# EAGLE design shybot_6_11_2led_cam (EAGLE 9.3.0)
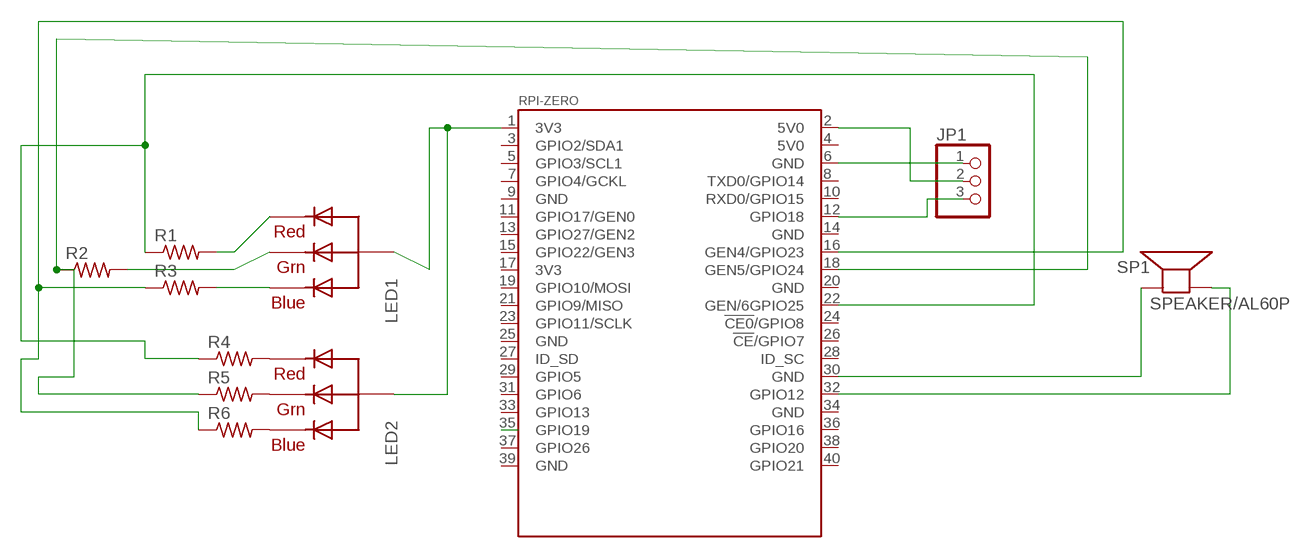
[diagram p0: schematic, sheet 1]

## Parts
JP1  PINHD-1X3  [1X03]
LED1  RGBLED_CA-5MM  [LED5MMRGB]
LED2  RGBLED_CA-5MM  [LED5MMRGB]
R1  R-US_0204/7  [0204/7]
R2  R-US_0204/7  [0204/7]
R3  R-US_0204/7  [0204/7]
R4  R-US_0204/7  [0204/7]
R5  R-US_0204/7  [0204/7]
R6  R-US_0204/7  [0204/7]
SP1  SPEAKER/AL60P  [AL60P]
U$1  RPI-ZERO  [RASPBERRYPI_BASTELSTUBE_V13_RASPI_BOARD_B+_FULL]

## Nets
3V3@1: LED1.2(VCC) LED2.2(VCC) U$1.1(3V3)
5V0@1: JP1.2 U$1.2(5V0)
GND@6: SP1.1(+) U$1.30(GND)
GND@8: JP1.1 U$1.6(GND)
N$1: JP1.3 U$1.12(GPIO18)
N$2: LED1.1(RED) R1.2
N$3: LED1.3(GREEN) R2.2
N$4: LED1.4(BLUE) R3.2
N$5: R2.1 R5.1 U$1.18(GEN5/GPIO24)
N$6: R1.1 R4.1 U$1.22(GEN/6GPIO25)
N$7: R3.1 R6.1 U$1.16(GEN4/GPIO23)
N$8: SP1.2(-) U$1.32(GPIO12)
N$9: LED2.1(RED) R4.2
N$10: U$1.35(GPIO19)
N$11: LED2.3(GREEN) R5.2
N$12: LED2.4(BLUE) R6.2
Unconnected: U$1.3(GPIO2/SDA1) U$1.4(5V0) U$1.5(GPIO3/SCL1) U$1.7(GPIO4/GCKL) U$1.8(TXD0/GPIO14) U$1.9(GND) U$1.10(RXD0/GPIO15) U$1.11(GPIO17/GEN0) U$1.13(GPIO27/GEN2) U$1.14(GND) U$1.15(GPIO22/GEN3) U$1.17(3V3) U$1.19(GPIO10/MOSI) U$1.20(GND) U$1.21(GPIO9/MISO) U$1.23(GPIO11/SCLK) U$1.24(!CE0!/GPIO8) U$1.25(GND) U$1.26(!CE!/GPIO7) U$1.27(ID_SD) U$1.28(ID_SC) U$1.29(GPIO5) U$1.31(GPIO6) U$1.33(GPIO13) U$1.34(GND) U$1.36(GPIO16) U$1.37(GPIO26) U$1.38(GPIO20) U$1.39(GND) U$1.40(GPIO21)

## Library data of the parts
JP1 = pinhead:PINHD-1X3: PIN HEADER
LED1 LED2 = adafruit:RGBLED_CA: RGB LED, common-anode 5MM Staggered pins 5mm Piranha package http://www.ladyada.net/library/pcb/eaglelibrary.html
R1-R6 = adafruit:R-US_: RESISTOR, American symbol
SP1 = adafruit:SPEAKER: SPEAKER
U$1 = RPI-Zero:RPI-ZERO

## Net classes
0 default: width 0.381 mm, drill 0.533 mm, clearance 0.406 mm

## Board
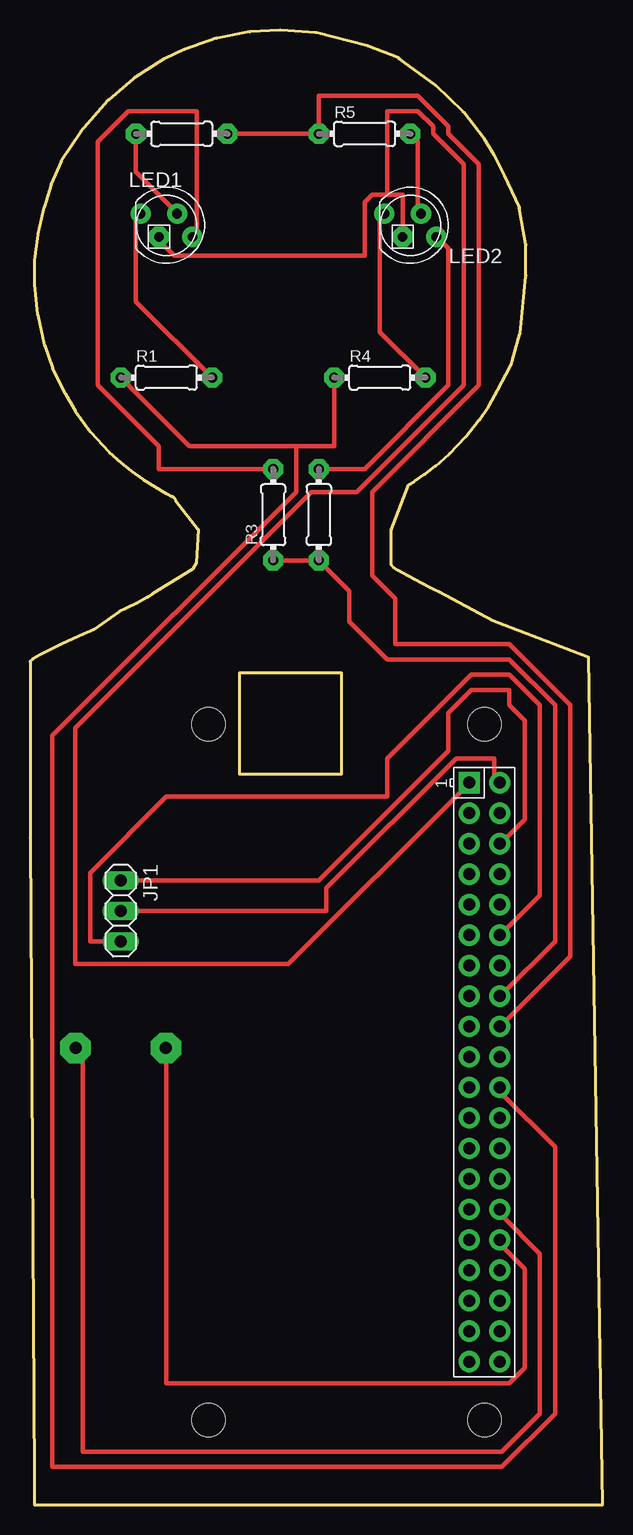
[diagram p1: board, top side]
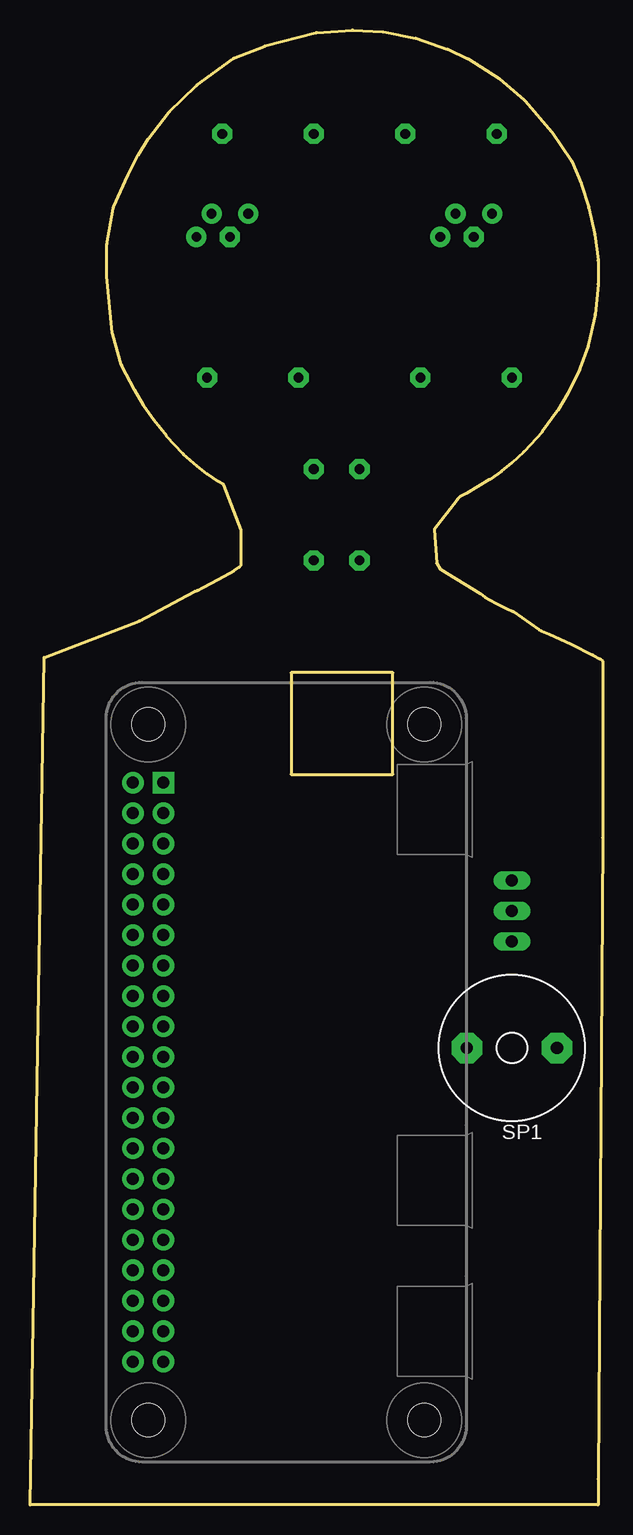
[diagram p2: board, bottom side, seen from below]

Size 47.72 x 122.96 mm. Coordinates in mm from the lower left corner, seen from the top.
Outline: 126 segments
Copper layers (1*16): Top 0.035mm / dielectric 1.5mm / Bottom 0.035mm
Design rules "default": minimum track width 6mil, minimum drill 0.35mm, track to track 6mil, track to pad 6mil, pad to pad 6mil, via to via 6mil, smd to smd 6mil, copper to edge 40mil, drill to drill 6mil, minimum pad ring 10mil, minimum via ring 8mil, stop-mask expansion 4mil, vias tented up to drill 0mil, thermal gap 10mil

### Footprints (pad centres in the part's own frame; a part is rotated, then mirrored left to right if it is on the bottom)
1X03 = drill 1.016 long: 1 -2.54,0; 2 0,0; 3 2.54,0
LED5MMRGB = drill 0.8 pad 1.676: 1 -2.159,0.968; 3 0.889,0.968; 4 2.159,-0.968 | drill 0.8 pad 1.676 octagon: 2 -0.635,-0.968
0204/7 = drill 0.813 pad 1.676 octagon: 1 -3.81,0; 2 3.81,0
AL60P = drill 1.016 pad 2.54 octagon: 1 -3.759,0; 2 3.759,0
RASPBERRYPI_BASTELSTUBE_V13_RASPI_BOARD_B+_FULL = drill 1 pad 1.778 square: 1 8.37,25.23 | drill 1 pad 1.778: 2 8.37,27.77; 3 10.91,25.23; 4 10.91,27.77; 5 13.45,25.23; 6 13.45,27.77; 7 15.99,25.23; 8 15.99,27.77; 9 18.53,25.23; 10 18.53,27.77; 11 21.07,25.23; 12 21.07,27.77; 13 23.61,25.23; 14 23.61,27.77; 15 26.15,25.23; 16 26.15,27.77; 17 28.69,25.23; 18 28.69,27.77; 19 31.23,25.23; 20 31.23,27.77; 21 33.77,25.23; 22 33.77,27.77; 23 36.31,25.23; 24 36.31,27.77; 25 38.85,25.23; 26 38.85,27.77; 27 41.39,25.23; 28 41.39,27.77; 29 43.93,25.23; 30 43.93,27.77; 31 46.47,25.23; 32 46.47,27.77; 33 49.01,25.23; 34 49.01,27.77; 35 51.55,25.23; 36 51.55,27.77; 37 54.09,25.23; 38 54.09,27.77; 39 56.63,25.23; 40 56.63,27.77 | hole 2.75: 3.5,3.5; 3.5,26.5; 61.5,3.5; 61.5,26.5

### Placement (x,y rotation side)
JP1  7.56,49.53 270 top
LED1  11.37,106.68 0 top
LED2  31.69,106.68 0 top
R1  11.37,93.98 0 top
R2  12.64,114.3 180 top
R3  20.26,82.55 90 top
R4  29.15,93.98 0 top
R5  27.88,114.3 0 top
R6  24.07,82.55 90 top
SP1  7.56,38.1 180 bottom
U$1  11.37,68.58 270 top

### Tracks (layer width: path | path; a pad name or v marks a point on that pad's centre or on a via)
3V3@1
  Top 0.381: 29.79,109.22 31.06,109.22 LED2.2 | 29.79,109.22 28.52,109.22 27.88,108.58 27.88,104.14 12.01,104.14 10.74,105.41 LED1.2 | 29.79,109.22 29.79,116.2 31.69,116.2 32.33,116.2 33.6,114.94 33.6,114.3 36.14,111.76 36.14,93.34 27.25,84.45 23.44,84.45 3.75,64.77 3.75,45.09 21.53,45.09 36.14,59.69 U$1.1
5V0@1
  Top 0.381: JP1.2 24.71,49.53 24.71,51.44 35.5,62.23 38.68,62.23 38.68,60.33 U$1.2
GND@6
  Top 0.381: U$1.30 39.31,24.13 42.49,20.95 42.49,7.62 39.31,4.45 4.39,4.45 4.39,38.1 SP1.1
GND@8
  Top 0.381: JP1.1 24.07,52.07 34.87,62.87 34.87,66.04 36.77,67.94 39.95,67.94 39.95,66.67 41.22,65.41 41.22,57.15 39.31,55.24 U$1.6
N$1
  Top 0.381: JP1.3 5.02,46.99 5.02,52.7 11.37,59.05 29.79,59.05 29.79,62.23 36.77,69.22 39.95,69.22 42.49,66.67 42.49,50.8 39.31,47.62 U$1.12
N$2
  Top 0.381: R1.2 8.83,100.33 8.83,107.31 LED1.1
N$3
  Top 0.381: R2.2 8.83,111.12 12.01,107.95 LED1.3
N$4
  Top 0.381: R3.2 10.74,86.36 10.74,88.27 5.66,93.34 5.66,113.67 8.2,116.2 13.91,116.2 13.91,106.05 LED1.4
N$5
  Top 0.381: R2.1 R5.1 24.07,117.47 32.33,117.47 34.87,114.94 34.87,114.78 34.87,114.3 37.41,111.76 37.41,93.34 28.52,84.45 28.52,77.47 30.42,75.56 30.42,71.75 39.95,71.75 45.03,66.67 45.03,45.72 39.31,40.01 U$1.18
N$6
  Top 0.381: R1.1 13.28,88.27 22.17,88.27 | 22.17,88.27 25.34,88.27 R4.1 | 22.17,88.27 22.17,84.45 1.85,64.14 1.85,3.17 39.31,3.17 43.76,7.62 43.76,29.84 39.31,34.29 U$1.22
N$7
  Top 0.381: R3.1 R6.1 26.61,76.2 26.61,73.66 29.79,70.48 39.95,70.48 43.76,66.67 43.76,46.99 39.31,42.55 U$1.16
N$8
  Top 0.381: U$1.32 39.31,21.59 41.22,19.68 41.22,11.43 39.95,10.16 11.37,10.16 11.37,38.1 SP1.2
N$9
  Top 0.381: R4.2 29.15,97.79 29.15,107.31 LED2.1
N$11
  Top 0.381: R5.2 32.33,113.67 32.33,107.95 LED2.3
N$12
  Top 0.381: R6.2 27.88,86.36 34.87,93.34 34.87,104.78 34.23,105.41 LED2.4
